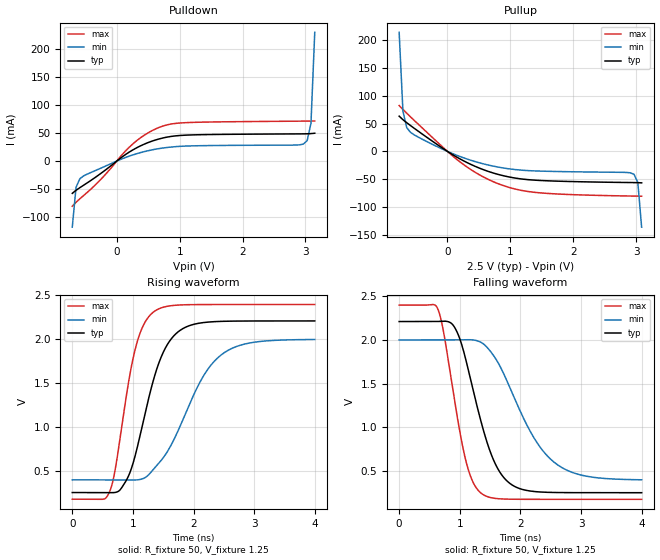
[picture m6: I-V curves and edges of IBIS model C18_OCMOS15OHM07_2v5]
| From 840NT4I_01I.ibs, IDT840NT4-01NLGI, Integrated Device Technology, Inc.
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| 3.25758e+00   -6.91296e-03   -1.23527e+00   -1.06037e-03
| 3.33333e+00   -4.29412e-02   -2.23636e+00   -4.10808e-03
| 3.40909e+00   -5.86126e-01   -3.23814e+00   -1.02850e-02
| 3.48485e+00   -1.79016e+00   -4.24043e+00   -2.01150e-02
| 3.56061e+00   -2.99494e+00   -5.24308e+00   -7.86962e-02
| 3.63636e+00   -4.20023e+00   -6.24601e+00   -1.11368e+00
| 3.71212e+00   -5.40589e+00   -7.24916e+00   -2.65554e+00
| 3.78788e+00   -6.61181e+00   -8.25246e+00   -4.19781e+00
| 3.86364e+00   -7.81791e+00   -9.25587e+00   -5.74033e+00
| 3.93939e+00   -9.02411e+00   -1.02593e+01   -7.28298e+00
| 4.01515e+00   -1.02304e+01   -1.12629e+01   -8.82566e+00
| 4.09091e+00   -1.14366e+01   -1.22664e+01   -1.03683e+01
| 4.16667e+00   -1.26429e+01   -1.32699e+01   -1.19109e+01
| 4.24242e+00   -1.38491e+01   -1.42735e+01   -1.34534e+01
| 4.31818e+00   -1.50552e+01   -1.52769e+01   -1.49957e+01
| 4.39394e+00   -1.62612e+01   -1.62803e+01   -1.65379e+01
| 4.46970e+00   -1.74672e+01   -1.72837e+01   -1.80798e+01
| 4.54545e+00   -1.86730e+01   -1.82870e+01   -1.96216e+01
| 4.62121e+00   -1.98787e+01   -1.92902e+01   -2.11633e+01
| 4.69697e+00   -2.10842e+01   -2.02933e+01   -2.27046e+01
| 4.77273e+00   -2.22897e+01   -2.12963e+01   -2.42458e+01
| 4.84848e+00   -2.34949e+01   -2.22993e+01   -2.57868e+01
| 4.92424e+00   -2.47001e+01   -2.33021e+01   -2.73276e+01
| 5.00000e+00   -2.59051e+01   -2.43049e+01   -2.88681e+01
[Model] C18_OCMOS15OHM07_2v5
Model_type   Output
Polarity   Non-Inverting
|   typ   min   max
C_comp   2pF   1.5pF   2.5pF
Vmeas = 1.25V
Rref = 50
Cref = 0
Vref = 1.25V
|   typ   min   max
[Voltage range]   2.5V   2.375V   2.625V
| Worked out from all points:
|   slope of the pulldown table from 0 to 0.375 V, typ, clamps not added: 13.9 ohm
|   slope of the pullup table from 0 to 0.375 V, typ, clamps not added: 15.9 ohm
|   rising waveform, R_fixture 50, V_fixture 1.25: 20-80 % time 453ps typ, 690ps min, 330ps max; typ from 0.256 V to 2.21 V
|   falling waveform, R_fixture 50, V_fixture 1.25: 20-80 % time 463ps typ, 707ps min, 332ps max; typ from 2.21 V to 0.256 V
[Pulldown]
|Voltage   I (typ)   I (min)   I (max)
|Note, modeling breaks down at 250mA and above.  This is well beyond the functional   |
|operating range of the device.  Should this scenario occur, catastrophic failure and   |
|possible damage to the device and/or board is of higher concern than the I-V curve   |
|behavior.  The IBIS checker will flag currents in excess of 10A with warnings.  Lines   |
|with currents in excess of 0.35 A have been commented out.  The points still remain|
|available to the user if the user desires to use them.   |
|-2.30000e+00   -2.48179e+01   -2.04013e+01   -2.98644e+01
|-2.10000e+00   -2.13531e+01   -1.78064e+01   -2.54360e+01
|-1.90000e+00   -1.78872e+01   -1.52107e+01   -2.10060e+01
|-1.70000e+00   -1.44201e+01   -1.26142e+01   -1.65742e+01
|-1.50000e+00   -1.09517e+01   -1.00170e+01   -1.21406e+01
|-1.49000e+00   -1.07783e+01   -9.88714e+00   -1.19189e+01
|-1.42977e+00   -9.73350e+00   -9.10489e+00   -1.05833e+01
|-1.36954e+00   -8.68862e+00   -8.32262e+00   -9.24752e+00
|-1.30931e+00   -7.64366e+00   -7.54033e+00   -7.91152e+00
|-1.24908e+00   -6.59862e+00   -6.75805e+00   -6.57533e+00
|-1.18885e+00   -5.55356e+00   -5.97580e+00   -5.23895e+00
|-1.12862e+00   -4.50851e+00   -5.19358e+00   -3.90244e+00
|-1.06839e+00   -3.46351e+00   -4.41144e+00   -2.56585e+00
|-1.00816e+00   -2.41864e+00   -3.62940e+00   -1.22927e+00
|-9.47931e-01   -1.37395e+00   -2.84751e+00   -2.18241e-01
|-8.87701e-01   -3.66354e-01   -2.06584e+00   -1.13641e-01
|-8.27471e-01   -9.83215e-02   -1.28447e+00   -9.85069e-02
|-7.67241e-01   -6.58945e-02   -5.03508e-01   -8.87035e-02
-707mV    -57.33mA   -117.4mA   -80.26mA
-646.8mV  -51.86mA   -46.44mA   -73.14mA
-586.6mV  -47.22mA   -31.34mA   -67mA
-225.2mV  -19.65mA   -11.23mA   -29.2mA
196.4mV   15.85mA    8.735mA    24.37mA
497.6mV   32.86mA    18.41mA    50.15mA
859mV     43.72mA    24.9mA     65.75mA
1.341V    46.9mA     27.36mA    69.12mA
2.967V    48.38mA    30.23mA    70.99mA
3.027V    48.5mA     36.38mA    71.05mA
3.087V    48.82mA    67.02mA    71.13mA
3.148V    49.5mA     228.8mA    71.27mA
| 3.20793e+00   5.06740e-02   8.68207e-01   7.16690e-02
| 3.26816e+00   5.31796e-02   1.62414e+00   7.25466e-02
| 3.32839e+00   6.52815e-02   2.38022e+00   7.39621e-02
| 3.38862e+00   1.66167e-01   3.13644e+00   7.58544e-02
| 3.44885e+00   8.87570e-01   3.89278e+00   7.82342e-02
| 3.50908e+00   1.89733e+00   4.64925e+00   8.25422e-02
| 3.56931e+00   2.90728e+00   5.40584e+00   1.15417e-01
| 3.62954e+00   3.91740e+00   6.16253e+00   6.39439e-01
| 3.68977e+00   4.92769e+00   6.91933e+00   1.93109e+00
| 3.75000e+00   5.93812e+00   7.67623e+00   3.22297e+00
| 3.76000e+00   6.10590e+00   7.80191e+00   3.43748e+00
| 4.00800e+00   1.02679e+01   1.09196e+01   8.75897e+00
| 4.25600e+00   1.44321e+01   1.40391e+01   1.40832e+01
| 4.50400e+00   1.85984e+01   1.71606e+01   1.94098e+01
| 4.75200e+00   2.27672e+01   2.02846e+01   2.47392e+01
| 5.00000e+00   2.69391e+01   2.34121e+01   3.00718e+01
[Pullup]
|Voltage   I (typ)   I (min)   I (max)
|Note, modeling breaks down at 250mA and above.  This is well beyond the functional   |
|operating range of the device.  Should this scenario occur, catastrophic failure and   |
|possible damage to the device and/or board is of higher concern than the I-V curve   |
|behavior.  The IBIS checker will flag currents in excess of 10A with warnings.  Lines   |
|with currents in excess of 0.35 A have been commented out.  The points still remain|
|available to the user if the user desires to use them.   |
|-2.30000e+00   2.36669e+01   1.93985e+01   2.85542e+01
|-2.10000e+00   2.02929e+01   1.68688e+01   2.42432e+01
|-1.90000e+00   1.69213e+01   1.43416e+01   1.99347e+01
|-1.70000e+00   1.35517e+01   1.18163e+01   1.56282e+01
|-1.50000e+00   1.01838e+01   9.29274e+00   1.13232e+01
|-1.49000e+00   1.00154e+01   9.16660e+00   1.11080e+01
|-1.42977e+00   9.00148e+00   8.40693e+00   9.81177e+00
|-1.36954e+00   7.98763e+00   7.64738e+00   8.51568e+00
|-1.30931e+00   6.97389e+00   6.88793e+00   7.21968e+00
|-1.24908e+00   5.96025e+00   6.12859e+00   5.92378e+00
|-1.18885e+00   4.94670e+00   5.36936e+00   4.62795e+00
|-1.12862e+00   3.93325e+00   4.61022e+00   3.33221e+00
|-1.06839e+00   2.91988e+00   3.85118e+00   2.03654e+00
|-1.00816e+00   1.90661e+00   3.09222e+00   7.40957e-01
|-9.47931e-01   8.93429e-01   2.33336e+00   1.41398e-01
|-8.87701e-01   1.80137e-01   1.57460e+00   9.85773e-02
|-8.27471e-01   7.89376e-02   8.15924e-01   8.94550e-02
-767.2mV  63.38mA    214.1mA    82.32mA
-707mV    56.91mA    72.22mA    75.4mA
-646.8mV  51.53mA    42.74mA    68.62mA
-586.6mV  46.39mA    34.17mA    62mA
256.7mV   -17mA      -11.58mA   -23.7mA
557.8mV   -32.31mA   -22.04mA   -45.17mA
859mV     -42.98mA   -29.32mA   -60.35mA
1.461V    -52.24mA   -35.44mA   -74.48mA
2.907V    -56.05mA   -38.52mA   -80.31mA
2.967V    -56.15mA   -41.36mA   -80.43mA
3.027V    -56.29mA   -56.07mA   -80.53mA
3.087V    -56.62mA   -136.3mA   -80.65mA
| 3.14770e+00   -5.74646e-02   -5.76910e-01   -8.08051e-02
| 3.20793e+00   -5.95007e-02   -1.35614e+00   -8.11736e-02
| 3.26816e+00   -6.51332e-02   -2.13596e+00   -8.22386e-02
| 3.32839e+00   -9.58634e-02   -2.91624e+00   -8.48263e-02
| 3.38862e+00   -3.71022e-01   -3.69687e+00   -8.94157e-02
| 3.44885e+00   -1.38204e+00   -4.47777e+00   -9.59588e-02
| 3.50908e+00   -2.42499e+00   -5.25889e+00   -1.07609e-01
| 3.56931e+00   -3.46836e+00   -6.04017e+00   -1.94606e-01
| 3.62954e+00   -4.51204e+00   -6.82159e+00   -1.14021e+00
| 3.68977e+00   -5.55595e+00   -7.60311e+00   -2.47520e+00
| 3.75000e+00   -6.60005e+00   -8.38473e+00   -3.81050e+00
| 3.76000e+00   -6.77342e+00   -8.51450e+00   -4.03222e+00
| 4.00800e+00   -1.10736e+01   -1.17334e+01   -9.53185e+00
| 4.25600e+00   -1.53741e+01   -1.49524e+01   -1.50315e+01
| 4.50400e+00   -1.96739e+01   -1.81710e+01   -2.05297e+01
| 4.75200e+00   -2.39726e+01   -2.13890e+01   -2.60264e+01
| 5.00000e+00   -2.82700e+01   -2.46061e+01   -3.15215e+01
[Ramp]
|   typ   min   max
dV/dt_r   1.17/0.452n   0.958/0.69n   1.328/0.33n
dV/dt_f   1.172/0.463n   0.957/0.707n   1.332/0.333n
R_load =   50.0000
[Rising Waveform]
R_fixture = 50
V_fixture = 1.25   |Vcc_typ
V_fixture_min = 1.1875 |Vcc_min
V_fixture_max = 1.3125 |Vcc_max
C_fixture = 0.0p
| Time   typ   min   max
0s        256.2mV    400.4mV    180.6mV
616.6ps   255.6mV    400.4mV    267.1mV
804.8ps   300.6mV    400.5mV    951.9mV
1.029ns   653.2mV    398.6mV    1.86V
1.333ns   1.522V     515.3mV    2.305V
1.514ns   1.868V     664.3mV    2.365V
1.722ns   2.069V     922.9mV    2.386V
2.13ns    2.185V     1.541V     2.393V
2.446ns   2.201V     1.815V     2.393V
4ns       2.207V     1.996V     2.393V
[Falling Waveform]
R_fixture = 50
V_fixture = 1.25   |Vcc_typ
V_fixture_min = 1.1875 |Vcc_min
V_fixture_max = 1.3125 |Vcc_max
C_fixture = 0.0p
| Time   typ   min   max
0s        2.207V     1.997V     2.393V
636.6ps   2.207V     1.997V     2.351V
969ps     2.066V     1.997V     1.077V
1.149ns   1.633V     2V         500.3mV
1.353ns   1.06V      1.968V     250.2mV
1.558ns   627.7mV    1.819V     193.9mV
1.77ns    395.9mV    1.544V     182.9mV
2.186ns   272.9mV    925.9mV    180.6mV
2.535ns   258.9mV    616.1mV    180.6mV
4ns       256.2mV    403.3mV    180.6mV
